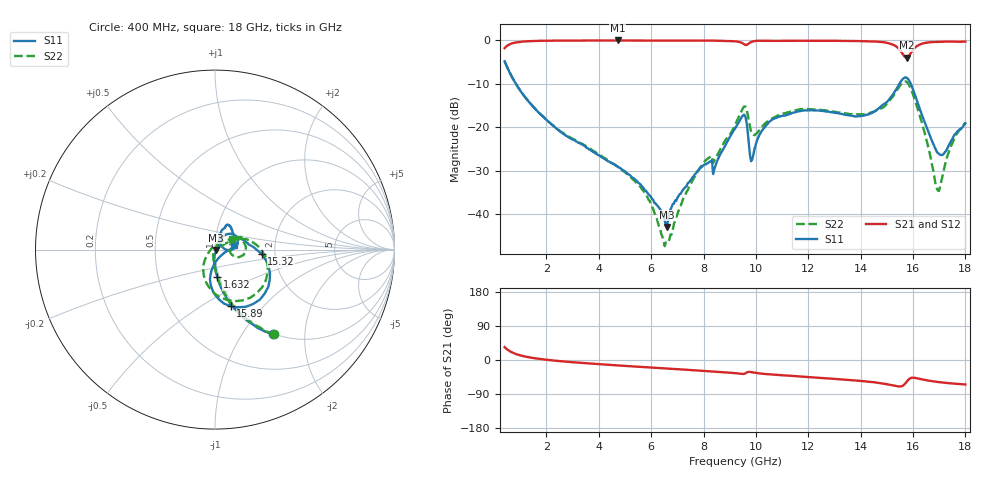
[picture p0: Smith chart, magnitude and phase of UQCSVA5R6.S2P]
!  Part Number  UQCSVA5R6  Mounting Orientation: Horizontal
!  Description: Ultra Low ESR Microwave capacitors
!  Application: Coupling, Bypass, Tuning, DC Block
!  Filters, Matching
# GHZ S DB R 50
! Freq  |S11|  S11 Ph  |S21|  S21 Ph  |S12|  S12 Ph  |S22|  S22 Ph
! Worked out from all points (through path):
!   401 points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, 400 MHz to 18 GHz, reference 50 ohm
!   highest |S21| = -0.04 dB at 4.712 GHz (marker M1); lowest = -4.0 dB at 15.76 GHz (marker M2)
!   group delay of S21, straight-line fit = 12.1 ps
!   lowest |S11| = -43.0 dB at 6.604 GHz (marker M3), VSWR 1.01, Z = 50.7 - j0.152 ohm
!   |S11| at or under -10 dB: 827 MHz to 15.48 GHz (14.66 GHz wide, 180 % of centre); 15.91 GHz to end of sweep
!   |S22| runs from -47.4 to -4.8 dB; largest |S21 - S12| = 0.0069
!   S11 on the Smith chart (normalised r, x): 400 MHz: 0.99, -1.39; 1.632 GHz: 0.98, -0.31; 15.32 GHz: 1.70, -0.09; 15.89 GHz: 0.96, -0.68; 18 GHz: 1.24, +0.06
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0.4  -4.84 -55.6  -1.81 34.0  -1.81 34.0  -4.80 -55.0
1.632  -16.19 -85.2  -0.14 3.8  -0.14 3.7  -16.20 -85.0
3.348  -23.92 -94.8  -0.07 -7.7  -0.06 -7.7  -23.82 -95.4
4.712  -29.04 -94.8  -0.04 -14.3  -0.03 -14.3  -29.09 -105.8
5.636  -33.59 -86.5  -0.05 -18.3  -0.04 -18.4  -34.21 -118.1
6.296  -38.58 -56.8  -0.05 -21.2  -0.05 -21.2  -42.80 -135.7
6.604  -42.99 -12.2  -0.08 -22.6  -0.06 -22.6  -46.69 169.8
7.66  -30.89 39.7  -0.07 -27.1  -0.06 -27.1  -31.38 64.8
8.452  -28.91 66.0  -0.09 -30.8  -0.07 -30.7  -27.24 26.0
9.2  -20.31 56.1  -0.24 -34.8  -0.23 -34.8  -19.53 30.6
9.552  -17.11 25.5  -0.93 -36.4  -0.91 -36.4  -15.26 6.1
9.86  -27.43 46.6  -0.30 -32.3  -0.29 -32.4  -21.61 -6.4
10.564  -18.52 69.3  -0.13 -38.2  -0.12 -38.1  -18.20 25.1
12.148  -16.10 59.8  -0.12 -45.8  -0.11 -45.8  -15.92 25.1
14.04  -17.38 35.3  -0.20 -55.5  -0.18 -55.5  -17.02 27.4
15.096  -13.57 4.8  -0.73 -65.0  -0.71 -65.0  -13.92 14.5
15.316  -11.66 -5.4  -1.27 -68.1  -1.24 -67.9  -12.22 3.2
15.756  -8.64 -55.2  -3.98 -57.3  -3.96 -57.3  -9.56 -53.7
15.888  -9.68 -74.3  -3.16 -48.5  -3.12 -48.4  -10.81 -76.7
16.944  -25.96 -64.9  -0.34 -58.0  -0.34 -57.9  -34.55 138.8
17.516  -22.56 -3.3  -0.29 -62.1  -0.29 -62.0  -23.50 45.6
18  -19.11 13.4  -0.30 -64.6  -0.29 -64.5  -18.96 31.5
